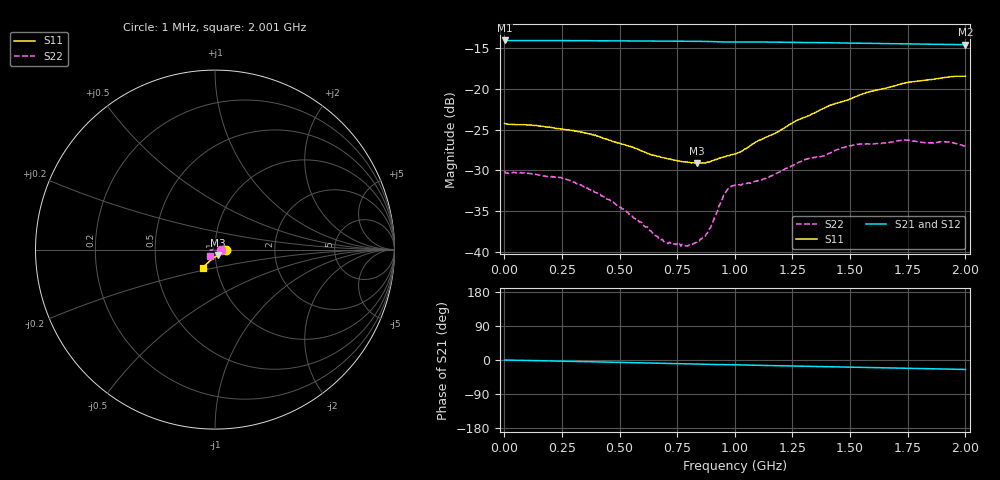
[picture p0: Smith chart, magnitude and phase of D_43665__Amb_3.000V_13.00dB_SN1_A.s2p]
! device id: 43665_
! dir: \\malibu\benchdata\1_engineers\tn_data\43665_75ohm\new\sparar\43665_\amb\3p000v\13p00db
! Serial: 1
! Insertion: A
! Temp: Amb
! VDD: 3.000V
! Attenuation Step: 13.00dB
! IDD: 1.450989e+00mA
! FILE NAME
! DATE 03-27-2009 08:36:33
! CORRECTED  DATA
#  Hz  S  RI  R  75
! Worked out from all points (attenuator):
!   401 points, 1 MHz to 2.001 GHz, reference 75 ohm
!   highest |S21| = -14.02 dB at 1 MHz (marker M1); lowest = -14.5 dB at 2.001 GHz (marker M2)
!   lowest |S11| = -29.1 dB at 836 MHz (marker M3), VSWR 1.07, Z = 77.6 - j4.66 ohm
!   |S11| at or under -10 dB: start of sweep to end of sweep
!   |S22| runs from -39.3 to -26.3 dB; largest |S21 - S12| = 0.00062
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1000000  0.0615 -0.000761  0.1992 -0.000356  0.1992 -0.000247  0.0311 -0.000353
2.36e8  0.0569 -0.00604  0.1985 -0.0101  0.1986 -0.0101  0.0267 0.0102
3.36e8  0.0537 -0.00909  0.1981 -0.0144  0.1981 -0.0144  0.0216 0.0135
5.16e8  0.0431 -0.0152  0.1969 -0.0224  0.197 -0.0224  0.0115 0.0142
6.71e8  0.0317 -0.0219  0.1955 -0.0291  0.1955 -0.029  0.000843 0.0119
7.01e8  0.0294 -0.0233  0.1952 -0.0304  0.1952 -0.0303  -0.000818 0.0114
7.91e8  0.0221 -0.0279  0.194 -0.0345  0.1941 -0.0345  -0.00726 0.00802
8.36e8  0.0181 -0.03  0.1934 -0.0366  0.1934 -0.0365  -0.0104 0.00468
8.71e8  0.0145 -0.0319  0.1927 -0.0384  0.1928 -0.0382  -0.0122 0.00179
8.91e8  0.0123 -0.0334  0.1922 -0.0393  0.1923 -0.0391  -0.0139 0.000125
9.61e8  0.00619 -0.038  0.1904 -0.0415  0.1905 -0.0413  -0.0231 -0.00216
9.81e8  0.00449 -0.039  0.1903 -0.042  0.1904 -0.0417  -0.0248 -0.00148
1.001e9  0.00225 -0.0398  0.1903 -0.0427  0.1904 -0.0425  -0.0255 -0.00131
1.126e9  -0.0101 -0.0489  0.1887 -0.0482  0.1889 -0.048  -0.027 -0.00766
1.336e9  -0.0295 -0.0639  0.1848 -0.0567  0.1852 -0.0565  -0.0314 -0.0211
1.381e9  -0.0339 -0.0675  0.1841 -0.0587  0.1844 -0.0586  -0.0305 -0.0239
1.506e9  -0.0435 -0.076  0.1811 -0.0632  0.1814 -0.0632  -0.0331 -0.0301
1.671e9  -0.054 -0.0873  0.1776 -0.069  0.1777 -0.0692  -0.0317 -0.0346
1.741e9  -0.0578 -0.0925  0.1759 -0.0713  0.1763 -0.0716  -0.0309 -0.0375
1.841e9  -0.0604 -0.0966  0.1737 -0.0743  0.1735 -0.0747  -0.0289 -0.0367
1.916e9  -0.0637 -0.0993  0.1721 -0.0766  0.1722 -0.0766  -0.029 -0.0373
2.001e9  -0.0644 -0.1012  0.1703 -0.079  0.17 -0.0795  -0.0259 -0.0359
